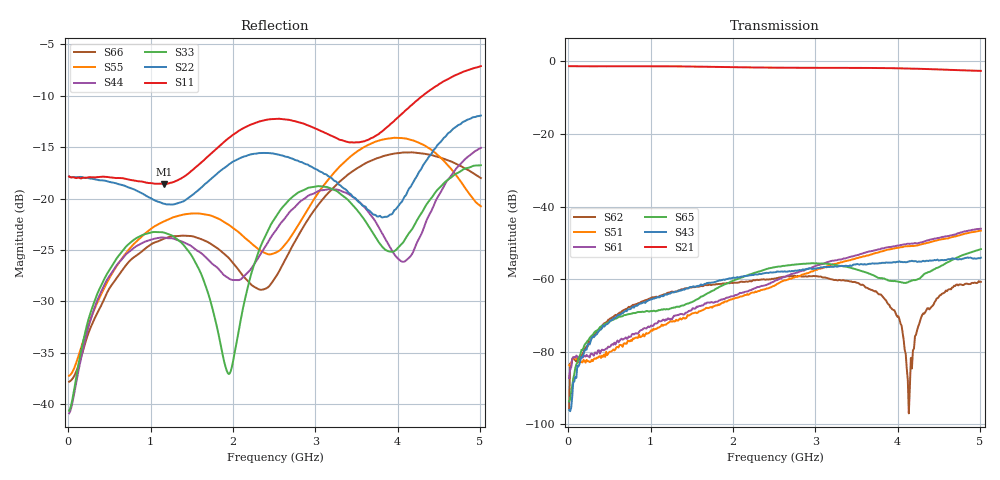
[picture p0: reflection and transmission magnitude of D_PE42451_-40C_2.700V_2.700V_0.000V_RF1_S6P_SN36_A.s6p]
! Device ID: PE42451
! Serial: 36
! Insertion: A
! Temp: -40C
! VDD: 2.700
! Control_Hi: 100.000
! Control_Lo: 0.000
! Logic State: RF1
! Port 1: RFC
! Port 2: RF1
! Port 3: RF2
! Port 4: RF3
! Port 5: RF4
! Port 6: RF5
! V1 = 2.70
! V2 = 0.00
! V3 = 0.00
! V4 = 0.00
! IDD: 1.070920e-05
#  Hz  S  RI  R  50
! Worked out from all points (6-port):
!   401 points, 10 MHz to 5.01 GHz, reference 50 ohm
!   strongest paths, dB at 10 MHz, 1.26 GHz, 2.51 GHz, 3.76 GHz, 5.01 GHz:
!     S21: -1.3, -1.4, -1.7, -1.8, -2.6
!     S43: -96.1, -63.6, -58.1, -55.7, -54.1
!     S65: -93.7, -67.9, -56.7, -59.6, -51.7
!     S61: -87.2, -71.0, -60.4, -51.8, -46.1
!     S51: -83.7, -71.7, -61.7, -52.7, -46.6
!     S62: -95.7, -63.4, -59.8, -64.0, -60.8
!   lowest |S11| = -18.6 dB at 1.16 GHz (marker M1), VSWR 1.27, Z = 56.9 - j10.6 ohm
!   |S11| at or under -10 dB: start of sweep to 4.303 GHz
